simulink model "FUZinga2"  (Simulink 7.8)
settings: Solver=ode45  StartTime=0.0  StopTime=30  FixedStep=0.1  RelTol=1e-3
undefined symbols (not defined in the file or in its folder): deg, kg, m, N, s
libraries: mblibv1 x5, fuzblock x1

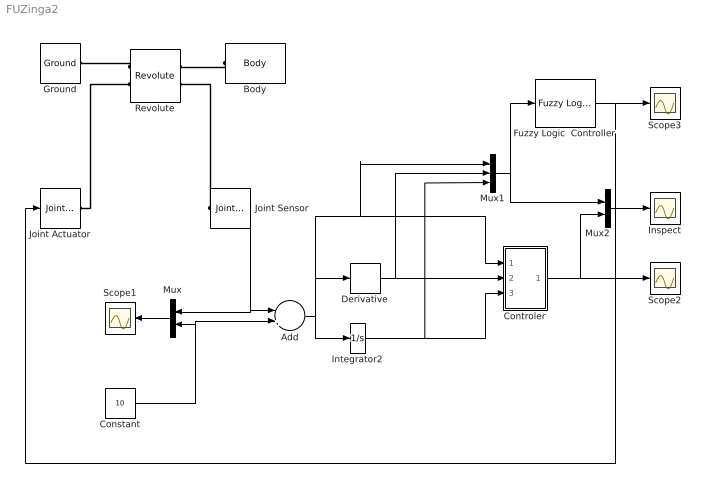
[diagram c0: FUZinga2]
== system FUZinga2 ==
  Add : Sum  Inputs=-+
  Body : mblibv1/Bodies/Body  LConnTagsString=CS1  UpdateFromCAD=off  DialogClass=MechanicalBodyBlock  Mass=1  MassUnits=kg  InertiaUnits=kg*m^2  Inertia=eye(3)  Shape=Cylinder  ShapeDims=[1 1]  ShapeUnits=m  ShapeUse=false  Density=1  DensityUnits=kg/m^3  DensityUse=false  GraphicsMode=MACHINE_DEFAULT  BodyColorSelMode=MACHINE_DEFAULT  BodyColor=[1 0 0]  AttachedToCS=CG  CG=Left$CG$[0 -0.5 0]$WORLD$WORLD$m$[0 0 0]$Euler X-Y-Z$deg$WORLD$false$none  WorkingFrames=Left$CS1$[0 0.5 0]$CG$CG$m$[0 0 0]$Euler X-Y-Z$deg$WORLD$true$none#Right$CS2$[0 -0.5 0]$CG$CG$m$[0 0 0]$Euler X-Y-Z$deg$WORLD$false$none  CGPos=[0 -0.5 0]  CGRot=[0 0 0]  CS0Pos=[]  CS0Rot=[]  CS1Pos=[0 0.5 0]  CS1Rot=[0 0 0]  CS2Pos=[0 -0.5 0]  CS2Rot=[0 0 0]  CS3Pos=[]  CS3Rot=[]  CS4Pos=[]  CS4Rot=[]  CS5Pos=[]  CS5Rot=[]  CS6Pos=[]  CS6Rot=[]  CS7Pos=[]  CS7Rot=[]  CS8Pos=[]  CS8Rot=[]  CS9Pos=[]  CS9Rot=[]  CS10Pos=[]  CS10Rot=[]  CS11Pos=[]  CS11Rot=[]  CS12Pos=[]  CS12Rot=[]  CS13Pos=[]  CS13Rot=[]  CS14Pos=[]  CS14Rot=[]  CS15Pos=[]  CS15Rot=[]  CS16Pos=[]  CS16Rot=[]  CS17Pos=[]  CS17Rot=[]  CS18Pos=[]  CS18Rot=[]  CS19Pos=[]  CS19Rot=[]  CS20Pos=[]  CS20Rot=[]
  Constant : Constant  Value=10
  Controler : Subsystem
  Derivative : Derivative
  Fuzzy Logic  Controller : fuzblock/Fuzzy Logic  Controller  fis=inga
  Ground : mblibv1/Bodies/Ground  UpdateFromCAD=off  LeftPortType=env  RightPortType=workingframe  PhysicalDomain=Mechanical  DialogClass=GroundBlock  CoordPosition=[0 0 0]  CoordPositionUnits=m  StateVectorMgrId=0  MachineId=[1 0]  ShowEnvPort=off
  Inspect : Scope
  Integrator2 : Integrator
  Joint Actuator : mblibv1/Sensors &  Actuators/Joint Actuator  UpdateFromCAD=off  PhysicalDomain=Mechanical  PortType=blob  ActuationStyle=Force  AngleUnits=deg  ArcVelocityUnits=deg/s  ArcAccelerationUnits=deg/s^2  CoordPositionUnits=m  VelocityUnits=m/s  AccelerationUnits=m/s^2  ForceUnits=N  TorqueUnits=N*m  ActiveIO=on  Width=1  DialogClass=MechanicalActuatorBlock  Primitive=R1  ReferenceFrame=Absolute (World)
  Joint Sensor : mblibv1/Sensors &  Actuators/Joint Sensor  UpdateFromCAD=off  PhysicalDomain=Mechanical  PortType=blob  Muxed=on  Pose=off  Angle=on  AngleUnits=deg  ArcVelocity=off  ArcVelocityUnits=deg/s  ArcAcceleration=off  ArcAccelerationUnits=deg/s^2  CoordPosition=on  CoordPositionUnits=m  Velocity=off  VelocityUnits=m/s  Acceleration=off  AccelerationUnits=m/s^2  Quaternion=on  QuaternionDT=off  QuaternionDDT=off  QuaternionUnits=off  OutputVector=[1]  ActiveIO=on  Width=1  DialogClass=MechanicalSensorBlock  Primitive=R1  Force=off  ForceUnits=N  Torque=off  TorqueUnits=N*m  ReferenceFrame=Absolute (World)  ReactionSensedSide=Base  ReactionReferenceFrame=Absolute (World)  ReactionForce=off  ReactionForceUnits=N  ReactionMoment=off  ReactionMomentUnits=N*m
  Mux : Mux  Inputs=2
  Mux1 : Mux  Inputs=3
  Mux2 : Mux  Inputs=2
  Revolute : mblibv1/Joints/Revolute  LConnTagsString=__newl0|SA1  RConnTagsString=__newr0|SA1  UpdateFromCAD=off  NumSAPorts=2  CutJoint=off  MarkAsCut=off  Primitives=prismatic  PrimitiveProps=R1$World$[0 0 1]$revolute  DialogClass=JointBlock  R1Axis=[0 0 1]
  Scope1 : Scope
  Scope2 : Scope
  Scope3 : Scope
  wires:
  Joint Sensor/1 -> Add/1, Mux/1
  Mux/1 -> Scope1/1
  Integrator2/1 -> Mux1/3, Controler/3(In3)
  Add/1 -> Derivative/1, Mux1/1, Controler/1(In1), Integrator2/1
  Derivative/1 -> Mux1/2, Controler/2(In2)
  Constant/1 -> Add/2, Mux/2
  Controler/1(Out1) -> Scope2/1, Mux2/2
  Mux1/1 -> Fuzzy Logic  Controller/1, Mux2/1
  Mux2/1 -> Inspect/1
  Fuzzy Logic  Controller/1 -> Scope3/1, Joint Actuator/1
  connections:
  Revolute/LConn1 -- Ground/RConn1
  Body/LConn1 -- Revolute/RConn1
  Joint Actuator/RConn1 -- Revolute/LConn2
  Joint Sensor/LConn1 -- Revolute/RConn2

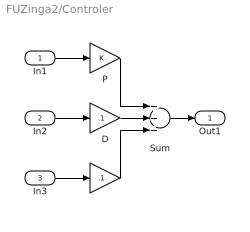
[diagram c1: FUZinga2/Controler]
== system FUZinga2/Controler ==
  In1 : Inport
  In2 : Inport  Port=2
  In3 : Inport  Port=3
  D : Gain  Gain=.1
  I : Gain  Gain=.1
  P : Gain
  Sum : Sum  Inputs=+++
  Out1 : Outport
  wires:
  I/1 -> Sum/3
  D/1 -> Sum/2
  P/1 -> Sum/1
  In1/1 -> P/1
  In2/1 -> D/1
  In3/1 -> I/1
  Sum/1 -> Out1/1
